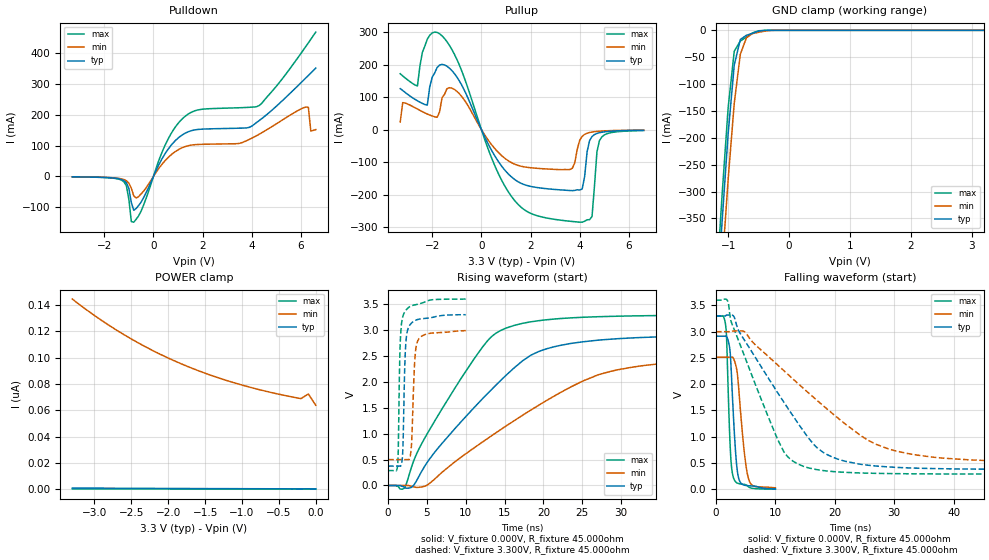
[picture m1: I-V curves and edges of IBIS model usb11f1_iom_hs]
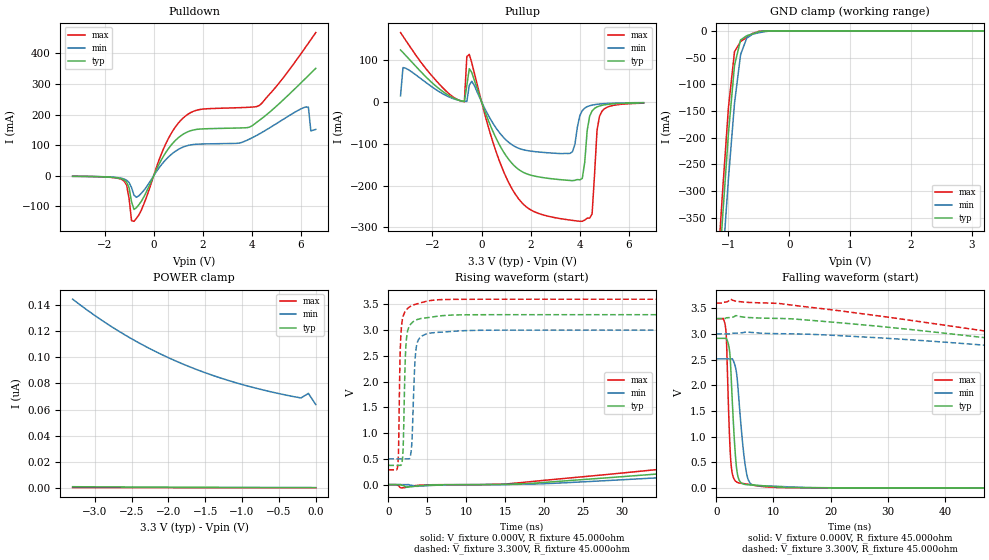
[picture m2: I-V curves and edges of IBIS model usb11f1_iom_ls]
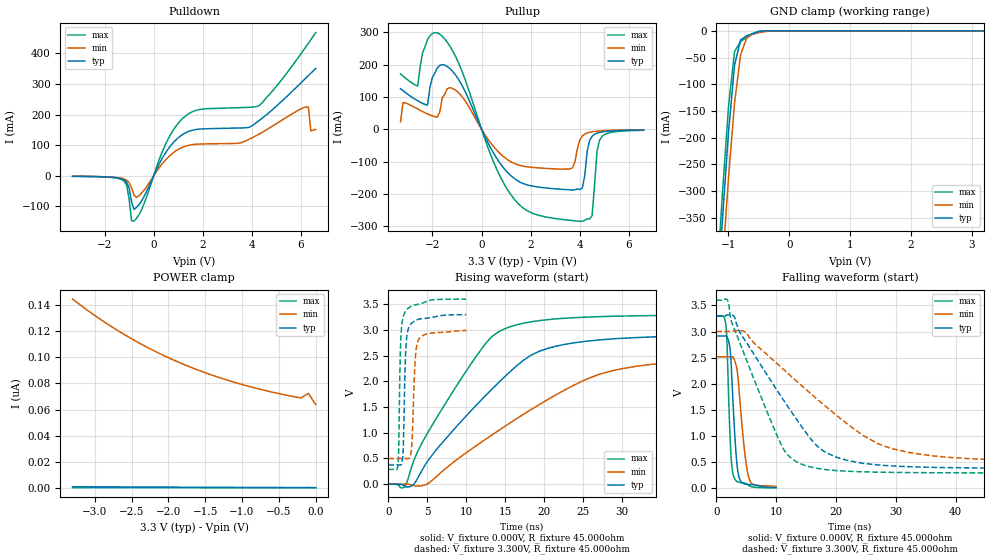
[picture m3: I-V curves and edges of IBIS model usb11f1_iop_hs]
[IBIS Ver]  4.0
[File Name]  lpc2929_lqfp144.ibs
[File Rev]  1.0
[Date]  Fri Oct 31 10:34:29 2008
[Source]  Package model is generic
[Notes]   IO models Rev 0.20 IBIS Model Design Automation Generation
[Copyright]  NXP Semiconductors 2008. All rights reserved.
[Disclaimer]
| NXP Semiconductors warrants and represents that the IBIS models
| identified herein are owned by NXP Semiconductors (NXP).  The
| models provided are not warranted as fully representing all of the
| operating characteristics and specifications of the semiconductor
| products to which the models relate.  Moreover, unless there is a
| signed, written agreement to the contrary, these models are furnished
| on an "as is" basis without support or warranty of any kind, either
| expressed or implied, regarding the use thereof, and NXP
| specifically disclaims all implied warranties of merchantability and
| fitness of the models for any purpose.
| NXP does not assume any liability arising out of the application
| or use of these IBIS models including infringement of patents and
| copyrights, nor does NXP convey any license under its patents and
| copyrights or the rights of others.
| NXP provides IBIS models as a service to our customers.  You and
| your company shall not distribute, convey, sell, or give these models
| to anyone else without receiving prior written permission from
| NXP.
[Component]   LPC29XX_LQFP144_01
[Manufacturer]  NXP
[Package]
|[Package Model]  LQFP144
|variable   typ   min   max
R_pkg   130.00m   123.00m   137.00m
L_pkg   8.30nH   7.50nH   9.20nH
C_pkg   1.00pF   0.80pF   1.30pF
| IMPORTANT NOTES:
| This model is valid for the following part types:
| LPC2929, LPC2927
| Signal names may be slightly different from the data
| sheet due to the 20 Char length limitation
[Pin]   signal_name   model_name   | comments
1 TDO bpats5thpept5v
2 P2.21 bpats5thpept5v
3 P0.24 bpats5thpept5v
4 P0.25 bpats5thpept5v
5 P0.26 bpats5thpept5v
6 P0.27 bpats5thpept5v
7 P0.28 bpats5thpept5v
8 P0.29 bpats5thpept5v
9 POWER_10 POWER
10 P2.22 bpats5thpept5v
11 P2.23 bpats5thpept5v
12 P3.6 bpats5thpept5v
13 P3.7 bpats5thpept5v
14 P0.30 bpats5thpept5v
15 P0.31 bpats5thpept5v
16 P2.24 bpats5thpept5v
17 P2.25 bpats5thpept5v
18 GND_21 POWER
19 USB1_IOP usb11f1_iop_ls
20 USB1_IOM usb11f1_iom_ls
21 POWER_26 POWER
22 POWER_27 POWER
23 GND_28 POWER
24 GND_30 POWER
25 P3_8 bpats5thpept5v
26 P3_9 bpats5thpept5v
27 P2_26 bpats5thpept5v
28 P2_27 bpats5thpept5v
29 P1.27 bpats5thpept5v
30 P1.26 bpats5thpept5v
31 POWER_48 POWER
32 P1.25 bpats5thpept5v
33 P1.24 bpats5thpept5v
34 P1.23 bpats5thpept5v
35 P1.22 bpats5thpept5v
36 TMS bpats5thpept5v
37 TCK bpats5thpept5v
38 P1.21 bpats5thpept5v
39 P1.20 bpats5thpept5v
40 P1.19 bpats5thpept5v
41 P1.18 bpats5thpept5v
42 P1.17 bpats5thpept5v
43 GNDE_62 POWER
44 P1.16 bpats5thpept5v
45 P2.0 bpats5thpept5v
46 P2.1 bpats5thpept5v
47 P3.10 bpats5thpept5v
48 P3.11 bpats5thpept5v
49 P1.15 bpats5thpept5v
50 P1.14 bpats5thpept5v
51 P1.13 bpats5thpept5v
52 P1.12 bpats5thpept5v
53 POWER_88 POWER
54 P2.2 bpats5thpept5v
55 P2.3 bpats5thpept5v
56 P1.11 bpats5thpept5v
57 P1.10 bpats5thpept5v
58 P3.12 bpats5thpept5v
59 GND_94 POWER
60 VDD_95 POWER
61 P3.13 bpats5thpept5v
62 P2.4 bpats5thpept5v
63 P2.5 bpats5thpept5v
64 P1.9 bpats5thpept5v
65 GNDE_100 POWER
66 P1.8 bpats5thpept5v
67 P1.7 bpats5thpept5v
68 P1.6 bpats5thpept5v
69 P2.6 bpats5thpept5v
70 P1.5 bpats5thpept5v
71 P1.4 bpats5thpept5v
72 TRSTN bpats5thpept5v
73 RSTN bpats5thpept5v
74 VSSA_OSC POWER
75 XOUT_OSC NC
76 XIN_OSC NC
77 VDDA_OSC POWER
78 VSSA_PLL POWER
79 P2.7 bpats5thpept5v
80 P3.14 bpats5thpept5v
81 P3.15 bpats5thpept5v
82 POWER_119 POWER
83 P2.8 bpats5thpept5v
84 P2.9 bpats5thpept5v
85 P1.3 bpats5thpept5v
86 P1.2 bpats5thpept5v
87 P1.1 bpats5thpept5v
88 GND_125 POWER
89 VDD_127 POWER
90 P1.0 bpats5thpept5v
91 P2.10 bpats5thpept5v
92 P2.11 bpats5thpept5v
93 P0.0 bpats5thpept5v
94 GNDE_134 POWER
95 P0.1 bpats5thpept5v
96 P0.2 bpats5thpept5v
97 P0.3 bpats5thpept5v
98 P3.0 bpats5thpept5v
99 P3.1 bpats5thpept5v
100 P2.12 bpats5thpept5v
101 P2.13 bpats5thpept5v
102 P0.4 bpats5thpept5v
103 P0.5 bpats5thpept5v
104 POWER_161 POWER
105 P0.6 bpats5thpept5v
106 P0.7 bpats5thpept5v
107 A3V3 POWER
108 JTAGSEL bpats5thpept5v
109 A5V POWER
110 VREFP NC
111 VREFN NC
112 P0.8 bpats5thpept5v
113 P0.9 bpats5thpept5v
114 P0.10 bpats5thpept5v
115 P0.11 bpats5thpept5v
116 P2.14 bpats5thpept5v
117 P2.15 bpats5thpept5v
118 P3.2 bpats5thpept5v
119 GNDE_178 POWER
120 P3.3 bpats5thpept5v
121 P0.12 bpats5thpept5v
122 P0.13 bpats5thpept5v
123 P0.14 bpats5thpept5v
124 P0.15 bpats5thpept5v
125 P0.16 bpats5thpept5v
126 P0.17 bpats5thpept5v
127 VDD_198 POWER
128 GND_199 POWER
129 P2.16 bpats5thpept5v
130 P2.17 bpats5thpept5v
131 POWER_202 POWER
132 P0.18 bpats5thpept5v
133 P0.19 bpats5thpept5v
134 P3.4 bpats5thpept5v
135 P3.5 bpats5thpept5v
136 P2.18 bpats5thpept5v
137 P2.19 bpats5thpept5v
138 P0.20 bpats5thpept5v
139 P0.21 bpats5thpept5v
140 P0.22 bpats5thpept5v
141 GNDE_212 POWER
142 P0.23 bpats5thpept5v
143 P2.20 bpats5thpept5v
144 TDI bpats5thpept5v
[Model Selector] bpats5thpept5v
bpats5thpept5v_p   Plain input Mode (p1=0, p2=1)
bpats5thpept5v_pd   Pull Down Mode   (p1=0, p2=0)
bpats5thpept5v_pu   Pull up   Mode   (p1=1, p2=1)
bpats5thpept5v_r   Repeater  Mode   (p1=1, p2=0)
[Model Selector] bpts5ptpht5v
bpts5ptpht5v_p_sh   Plain input Mode (p1=0, p2=1)
bpts5ptpht5v_p_sl   Plain input Mode (p1=0, p2=1)
bpts5ptpht5v_pd_sh   Pull Down Mode (p1=1, p2=1)
bpts5ptpht5v_pd_sl   Pull Down Mode (p1=1, p2=1)
bpts5ptpht5v_pu_sh   Pull Up Mode (p1=0, p2=0)
bpts5ptpht5v_pu_sl   Pull Up Mode (p1=0, p2=0)
bpts5ptpht5v_r_sh   Repeater Mode (p1=1, p2=0)
bpts5ptpht5v_r_sl   Repeater Mode (p1=1, p2=0)
| Models and submodels in the file (16): usb11f1_iom_hs (I/O), usb11f1_iom_ls (I/O), usb11f1_iop_hs (I/O), usb11f1_iop_ls (I/O), bpats5thpept5v_p (I/O), bpats5thpept5v_pd (I/O), bpats5thpept5v_pu (I/O), bpats5thpept5v_r (I/O), bpts5ptpht5v_p_sh (I/O), bpts5ptpht5v_p_sl (I/O), bpts5ptpht5v_pd_sh (I/O), bpts5ptpht5v_pd_sl (I/O), bpts5ptpht5v_pu_sh (I/O), bpts5ptpht5v_pu_sl (I/O), bpts5ptpht5v_r_sh (I/O), bpts5ptpht5v_r_sl (I/O)
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| usb11f1
|   Universal Serial Bus Pad
|   Revision 1.1 Specification
|   Programmable Single Ended Core Input
|   Forced Single Ended Low
|   Switchable between
|   - high speed output mode
|   - low speed output mode
|   - low/high speed input mode
| |   Rev 0.20 IBIS Model Design Automation Generation   |
| |   N O N - S I L I C O N   C O R R E L A T E D   |
| |   This IBIS [Model] is pre-Beta tactical support   |
| |  Note: this IBIS [Model] contains clamp curves generated   |
| |   through simulation which should not be relied upon   |
| Pccmos14 hliolib_nlm 4.0
|   0.18 um 3.3V pad library
|   six level metal
|   dual oxide
|   single threshold voltage
|   nominal line mixed supply
|   parasitic extracted netlists
| Process block c14
| High Speed Output Mode
[Model]   usb11f1_iom_hs | of usb11f1
Model_type   I/O
Polarity   Non-Inverting
Enable   Active-Low
|  Reciever Thresholds
Vinl   = 0.8V
Vinh   = 2.0V
| AC Test Load Conditions
Vref   = 0
Cref   = 0
Rref   = 1000000000
Vmeas   = 1.65
| [Process Range]   typical   min   max
| C_comp edge width   400.000ps   400.000ps   400.000ps
| C_comp Tstrobe   40.000fs   40.000fs   40.000fs
C_comp   3.752pF   3.496pF   4.045pF
[Temperature Range]   25   125   -40
[Voltage Range]   3.30V   3.00V   3.60V
[GND Clamp Reference]   0.00V   0.00V   0.00V
[Pulldown Reference]   0.00V   0.00V   0.00V
[POWER Clamp Reference]   3.30V   3.00V   3.60V
[Pullup Reference]   3.30V   3.00V   3.60V
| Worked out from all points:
|   slope of the pulldown table from 0 to 0.495 V, typ, clamps not added: 6.48 ohm
|   slope of the pullup table from 0 to 0.495 V, typ, clamps not added: 6.61 ohm
|   GND clamp passes 1 mA (typ) near -0.46 V on its own axis
|   rising waveform, V_fixture 0.000V, R_fixture 45.000ohm: 20-80 % time 11ns typ, 15.9ns min, 8.17ns max; typ from 0 V to 2.91 V
|   falling waveform, V_fixture 0.000V, R_fixture 45.000ohm: 20-80 % time 845ps typ, 1.21ns min, 607ps max; typ from 2.91 V to 0.006 V
|   rising waveform, V_fixture 3.300V, R_fixture 45.000ohm: 20-80 % time 320ps typ, 399ps min, 287ps max; typ from 0.374 V to 3.3 V
|   falling waveform, V_fixture 3.300V, R_fixture 45.000ohm: 20-80 % time 10.2ns typ, 15.5ns min, 6.95ns max; typ from 3.3 V to 0.374 V
[GND Clamp]
| ref voltage   0.00V   0.00V   0.00V
|   Voltage   I(typ)   I(min)   I(max)
-3.3V     -4.618A    -4.67A     -4.591A
-1.2V     -533.4mA   -616mA     -486.2mA
-1.1V     -356.1mA   -441.1mA   -306.9mA
-1V       -192.1mA   -277.1mA   -143.8mA
-900mV    -64.59mA   -135.6mA   -38.91mA
-800mV    -17.04mA   -44.51mA   -19.95mA
-700mV    -9.237mA   -13.86mA   -12.52mA
-600mV    -5.456mA   -6.064mA   -4.789mA
-500mV    -1.495mA   -3.666mA   -840.2uA
-300mV    -6.625uA   -179.7uA   -408.9nA
3.2V      293.2pA    68.89nA    105.6pA
[Power Clamp]   | Vtable = Vcc - Vpad
| ref voltage   3.30V   3.00V   3.60V
|   Voltage   I(typ)   I(min)   I(max)
-3.3V     1.005nA    144.5nA    354.7pA
-3V       911.2pA    132nA      335.1pA
-2.6V     800.8pA    117.4nA    309pA
-2.3V     727.5pA    108nA      289.6pA
-1.9V     640.7pA    97.15nA    263.8pA
-1.6V     582.9pA    90.25nA    244.5pA
-1.3V     530.6pA    84.3nA     225.3pA
-1V       483pA      79.18nA    206.1pA
-700mV    439.6pA    74.79nA    187pA
-200mV    377.6pA    68.89nA    155pA
-100mV    416.5pA    72.39nA    142.6pA
0V        319.1pA    63.83nA    125.6pA
[Pulldown]
| ref voltage   0.00V   0.00V   0.00V
|   Voltage   I(typ)   I(min)   I(max)
-3.3V     -1.652mA   -1.454mA   -1.796mA
-1.2V     -13.92mA   -10.45mA   -17.73mA
-1.1V     -21.12mA   -14.45mA   -30.61mA
-900mV    -85.23mA   -38.63mA   -146.6mA
-800mV    -110mA     -63.62mA   -148.7mA
500mV     77.03mA    53.28mA    105.7mA
1.1V      130.5mA    90.36mA    180.9mA
4.3V      181mA      136.8mA    229.8mA
6.2V      319.7mA    225.1mA    421.9mA
6.3V      327.6mA    224.1mA    433.3mA
6.4V      335.5mA    146.8mA    444.9mA
6.6V      351.2mA    151.8mA    468.2mA
[Pullup]   | Vtable = Vcc - Vpad
| ref voltage   3.30V   3.00V   3.60V
|   Voltage   I(typ)   I(min)   I(max)
-3.3V     125.8mA    23.2mA     171.5mA
-2.6V     88.3mA     62.98mA    134mA
-2.2V     74.98mA    47.7mA     277.9mA
-1.6V     200.3mA    97.67mA    288.3mA
-1V       161.8mA    117.7mA    216.4mA
900mV     -120mA     -85.3mA    -166.8mA
2.5V      -180.9mA   -120.7mA   -269.8mA
3.7V      -188.1mA   -119.1mA   -283mA
4.1V      -182.9mA   -20.96mA   -285.2mA
4.4V      -34.22mA   -9.287mA   -277.5mA
4.8V      -9.883mA   -5.195mA   -34.66mA
6.6V      -2.365mA   -1.804mA   -3.161mA
[Ramp]
R_load   = 60.000ohm
|   dV/dt(typ)   dV/dt(min)   dV/dt(max)
dV/dt_r   803.394mV/4.105ns   370.492mV/2.885ns   1.331V/4.905ns
dV/dt_f   843.371mV/4.620ns   360.067mV/3.240ns   1.540V/5.255ns
[Rising Waveform]  | cubic spline decimation from 16001 points
V_fixture   = 0.000V
R_fixture   = 45.000ohm
|   Time   V(typ)   V(min)   V(max)
0s        443.9pV    34.48nV    250.2pV
2.05ns    -28.68mV   9.864uV    -55.51mV
3.165ns   -16.71mV   -18.22mV   419.1mV
5.14ns    468.7mV    16.86mV    1.024V
12.03ns   1.653V     825.1mV    2.643V
16.32ns   2.281V     1.258V     3.093V
21.57ns   2.684V     1.741V     3.215V
26.99ns   2.804V     2.132V     3.257V
32.92ns   2.858V     2.315V     3.276V
80ns      2.912V     2.506V     3.295V
[Falling Waveform]  | cubic spline decimation from 2001 points
V_fixture   = 0.000V
R_fixture   = 45.000ohm
|   Time   V(typ)   V(min)   V(max)
0s        2.914V     2.514V     3.296V
1.65ns    2.919V     2.514V     3.102V
1.79ns    2.905V     2.514V     2.86V
2.415ns   2.567V     2.514V     760.7mV
2.935ns   1.397V     2.492V     222.4mV
3.365ns   607.8mV    2.348V     134.4mV
3.78ns    227.5mV    1.985V     109.9mV
4.655ns   81.21mV    824.9mV    94.37mV
5.45ns    66.93mV    210.5mV    47.53mV
10ns      6.197mV    27.24mV    1.84mV
[Rising Waveform]  | cubic spline decimation from 2001 points
V_fixture   = 3.300V
V_fixture_min = 3.000V
V_fixture_max = 3.600V
R_fixture   = 45.000ohm
|   Time   V(typ)   V(min)   V(max)
0s        373.7mV    499.4mV    287.7mV
1.215ns   373.7mV    499.4mV    375.2mV
1.575ns   374.2mV    499.5mV    2.78V
1.87ns    595mV      499.5mV    3.244V
2.065ns   1.779V     499.5mV    3.327V
2.355ns   2.862V     499.5mV    3.393V
2.96ns    3.126V     677.4mV    3.465V
3.43ns    3.18V      2.396V     3.486V
3.84ns    3.205V     2.798V     3.499V
10ns      3.296V     2.989V     3.598V
[Falling Waveform]  | cubic spline decimation from 16001 points
V_fixture   = 3.300V
V_fixture_min = 3.000V
V_fixture_max = 3.600V
R_fixture   = 45.000ohm
|   Time   V(typ)   V(min)   V(max)
0s        3.3V       3V         3.6V
1.96ns    3.316V     3V         3.585V
2.955ns   3.297V     3.013V     3.074V
4.81ns    2.836V     3V         2.532V
11.41ns   1.661V     2.26V      717.5mV
14.73ns   1.108V     1.92V      436.6mV
20.49ns   574.7mV    1.36V      330.4mV
25.63ns   457.1mV    931.8mV    306.2mV
31.99ns   408.5mV    686.3mV    295.4mV
80ns      374.5mV    503.6mV    287.9mV
| usb11f1
|   Universal Serial Bus Pad
|   Revision 1.1 Specification
|   Programmable Single Ended Core Input
|   Forced Single Ended Low
|   Switchable between
|   - high speed output mode
|   - low speed output mode
|   - low/high speed input mode
| |   Rev 0.20 IBIS Model Design Automation Generation   |
| |   N O N - S I L I C O N   C O R R E L A T E D   |
| |   This IBIS [Model] is pre-Beta tactical support   |
| |  Note: this IBIS [Model] contains clamp curves generated   |
| |   through simulation which should not be relied upon   |
| Pccmos14 hliolib_nlm 4.0
|   0.18 um 3.3V pad library
|   six level metal
|   dual oxide
|   single threshold voltage
|   nominal line mixed supply
|   parasitic extracted netlists
| Process block c14
| Low Speed Output Mode
[Model]   usb11f1_iom_ls | of usb11f1
Model_type   I/O
Polarity   Non-Inverting
Enable   Active-Low
|  Reciever Thresholds
Vinl   = 0.8V
Vinh   = 2.0V
| AC Test Load Conditions
Vref   = 0
Cref   = 0
Rref   = 1000000000
Vmeas   = 1.65
| [Process Range]   typical   min   max
| C_comp edge width   400.000ps   400.000ps   400.000ps
| C_comp Tstrobe   40.000fs   40.000fs   40.000fs
C_comp   3.752pF   3.496pF   4.045pF
[Temperature Range]   25   125   -40
[Voltage Range]   3.30V   3.00V   3.60V
[GND Clamp Reference]   0.00V   0.00V   0.00V
[Pulldown Reference]   0.00V   0.00V   0.00V
[POWER Clamp Reference]   3.30V   3.00V   3.60V
[Pullup Reference]   3.30V   3.00V   3.60V
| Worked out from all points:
|   slope of the pulldown table from 0 to 0.495 V, typ, clamps not added: 6.48 ohm
|   slope of the pullup table from 0 to 0.495 V, typ, clamps not added: 6.61 ohm
|   GND clamp passes 1 mA (typ) near -0.46 V on its own axis
|   rising waveform, V_fixture 0.000V, R_fixture 45.000ohm: 20-80 % time 151ns typ, 180ns min, 132ns max; typ from 0 V to 2.91 V
|   falling waveform, V_fixture 0.000V, R_fixture 45.000ohm: 20-80 % time 850ps typ, 1.23ns min, 609ps max; typ from 2.91 V to 0 V
|   rising waveform, V_fixture 3.300V, R_fixture 45.000ohm: 20-80 % time 318ps typ, 398ps min, 284ps max; typ from 0.374 V to 3.3 V
|   falling waveform, V_fixture 3.300V, R_fixture 45.000ohm: 20-80 % time 156ns typ, 194ns min, 133ns max; typ from 3.3 V to 0.38 V
[GND Clamp]
| ref voltage   0.00V   0.00V   0.00V
|   Voltage   I(typ)   I(min)   I(max)
-3.3V     -4.618A    -4.67A     -4.591A
-1.2V     -533.4mA   -616mA     -486.2mA
-1.1V     -356.1mA   -441.1mA   -306.9mA
-1V       -192.1mA   -277.1mA   -143.8mA
-900mV    -64.59mA   -135.6mA   -38.91mA
-800mV    -17.04mA   -44.51mA   -19.95mA
-700mV    -9.237mA   -13.86mA   -12.52mA
-600mV    -5.456mA   -6.064mA   -4.789mA
-500mV    -1.495mA   -3.666mA   -840.2uA
-300mV    -6.625uA   -179.7uA   -408.9nA
3.2V      293.2pA    68.89nA    105.6pA
[Power Clamp]   | Vtable = Vcc - Vpad
| ref voltage   3.30V   3.00V   3.60V
|   Voltage   I(typ)   I(min)   I(max)
-3.3V     1.005nA    144.5nA    354.7pA
-3V       911.2pA    132nA      335.1pA
-2.6V     800.8pA    117.4nA    309pA
-2.3V     727.5pA    108nA      289.6pA
-1.9V     640.7pA    97.15nA    263.8pA
-1.6V     582.9pA    90.25nA    244.5pA
-1.3V     530.6pA    84.3nA     225.3pA
-1V       483pA      79.18nA    206.1pA
-700mV    439.6pA    74.79nA    187pA
-200mV    377.6pA    68.89nA    155pA
-100mV    416.5pA    72.39nA    142.6pA
0V        319.1pA    63.83nA    125.6pA
[Pulldown]
| ref voltage   0.00V   0.00V   0.00V
|   Voltage   I(typ)   I(min)   I(max)
-3.3V     -1.652mA   -1.454mA   -1.796mA
-1.2V     -13.92mA   -10.45mA   -17.73mA
-1.1V     -21.12mA   -14.45mA   -30.61mA
-900mV    -85.23mA   -38.63mA   -146.6mA
-800mV    -110mA     -63.62mA   -148.7mA
500mV     77.03mA    53.28mA    105.7mA
1.1V      130.5mA    90.36mA    180.9mA
4.3V      181mA      136.8mA    229.8mA
6.2V      319.7mA    225.1mA    421.9mA
6.3V      327.6mA    224.1mA    433.3mA
6.4V      335.5mA    146.8mA    444.9mA
6.6V      351.2mA    151.8mA    468.2mA
[Pullup]   | Vtable = Vcc - Vpad
| ref voltage   3.30V   3.00V   3.60V
|   Voltage   I(typ)   I(min)   I(max)
-3.3V     123.9mA    14.28mA    165.4mA
-3.2V     117.8mA    81.84mA    156.7mA
-800mV    1.807mA    2.206mA    1.368mA
-500mV    79.1mA     39.57mA    113.5mA
1V        -129mA     -91.21mA   -180.1mA
2.5V      -180.9mA   -120.7mA   -269.8mA
3.7V      -188.1mA   -119.1mA   -283mA
4.1V      -182.9mA   -20.96mA   -285.2mA
4.4V      -34.22mA   -9.287mA   -277.5mA
4.5V      -21.68mA   -7.778mA   -267.6mA
4.8V      -9.883mA   -5.195mA   -34.66mA
6.6V      -2.365mA   -1.804mA   -3.161mA
[Ramp]
R_load   = 60.000ohm
|   dV/dt(typ)   dV/dt(min)   dV/dt(max)
dV/dt_r   621.133mV/49.000ns   449.857mV/47.650ns   797.798mV/50.350ns
dV/dt_f   625.100mV/49.850ns   419.096mV/47.300ns   836.278mV/52.000ns
[Rising Waveform]  | cubic spline decimation from 16001 points
V_fixture   = 0.000V
R_fixture   = 45.000ohm
|   Time   V(typ)   V(min)   V(max)
0s        443.9pV    34.49nV    250.2pV
1.75ns    -12.65mV   2.275uV    -62.94mV
15.6ns    5.793mV    2.484mV    18.34mV
130.2ns   1.408V     1.033V     1.795V
182.8ns   2.006V     1.49V      2.541V
215.3ns   2.324V     1.742V     2.891V
240.8ns   2.515V     1.918V     3.033V
308.5ns   2.738V     2.227V     3.184V
402.4ns   2.838V     2.384V     3.248V
800ns     2.907V     2.501V     3.292V
[Falling Waveform]  | cubic spline decimation from 2001 points
V_fixture   = 0.000V
R_fixture   = 45.000ohm
|   Time   V(typ)   V(min)   V(max)
0s        2.914V     2.514V     3.296V
1.65ns    2.918V     2.514V     3.099V
1.8ns     2.902V     2.514V     2.824V
2.25ns    2.726V     2.514V     1.203V
2.75ns    1.81V      2.518V     313.5mV
3.35ns    628.5mV    2.352V     134.1mV
3.85ns    197.5mV    1.878V     99.95mV
5.3ns     62.15mV    280.7mV    75.31mV
6.75ns    52.95mV    48.63mV    46.78mV
100ns     89.79uV    122.2uV    67.53uV
[Rising Waveform]  | cubic spline decimation from 2001 points
V_fixture   = 3.300V
V_fixture_min = 3.000V
V_fixture_max = 3.600V
R_fixture   = 45.000ohm
|   Time   V(typ)   V(min)   V(max)
0s        373.7mV    499.4mV    287.7mV
1.25ns    373.7mV    499.5mV    440.2mV
1.55ns    374.8mV    499.5mV    2.698V
1.85ns    558.6mV    499.5mV    3.237V
2.15ns    2.321V     499.5mV    3.356V
2.4ns     2.919V     499.6mV    3.406V
3ns       3.136V     762.4mV    3.473V
3.6ns     3.197V     2.674V     3.505V
4.85ns    3.237V     2.922V     3.556V
100ns     3.3V       3V         3.6V
[Falling Waveform]  | cubic spline decimation from 16001 points
V_fixture   = 3.300V
V_fixture_min = 3.000V
V_fixture_max = 3.600V
R_fixture   = 45.000ohm
|   Time   V(typ)   V(min)   V(max)
0s        3.3V       3V         3.6V
2.45ns    3.319V     3V         3.678V
28.5ns    3.148V     2.924V     3.35V
114.5ns   2.081V     2.172V     1.981V
188.3ns   1.259V     1.566V     937.8mV
232.7ns   858.8mV    1.248V     557.2mV
289.8ns   591.2mV    921.5mV    405.8mV
389.9ns   453.5mV    659.5mV    332.3mV
557.6ns   398mV      548.8mV    301.5mV
800ns     380mV      513mV      291.2mV
| usb11f1
|   Universal Serial Bus Pad
|   Revision 1.1 Specification
|   Programmable Single Ended Core Input
|   Forced Single Ended Low
|   Switchable between
|   - high speed output mode
|   - low speed output mode
|   - low/high speed input mode
| |   Rev 0.20 IBIS Model Design Automation Generation   |
| |   N O N - S I L I C O N   C O R R E L A T E D   |
| |   This IBIS [Model] is pre-Beta tactical support   |
| |  Note: this IBIS [Model] contains clamp curves generated   |
| |   through simulation which should not be relied upon   |
| Pccmos14 hliolib_nlm 4.0
|   0.18 um 3.3V pad library
|   six level metal
|   dual oxide
|   single threshold voltage
|   nominal line mixed supply
|   parasitic extracted netlists
| Process block c14
| High Speed Output Mode
[Model]   usb11f1_iop_hs | of usb11f1
Model_type   I/O
Polarity   Non-Inverting
Enable   Active-Low
|  Reciever Thresholds
Vinl   = 0.8V
Vinh   = 2.0V
| AC Test Load Conditions
Vref   = 0
Cref   = 0
Rref   = 1000000000
Vmeas   = 1.65
| [Process Range]   typical   min   max
| C_comp edge width   400.000ps   400.000ps   400.000ps
| C_comp Tstrobe   40.000fs   40.000fs   40.000fs
C_comp   3.752pF   3.496pF   4.045pF
[Temperature Range]   25   125   -40
[Voltage Range]   3.30V   3.00V   3.60V
[GND Clamp Reference]   0.00V   0.00V   0.00V
[Pulldown Reference]   0.00V   0.00V   0.00V
[POWER Clamp Reference]   3.30V   3.00V   3.60V
[Pullup Reference]   3.30V   3.00V   3.60V
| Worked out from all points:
|   slope of the pulldown table from 0 to 0.495 V, typ, clamps not added: 6.48 ohm
|   slope of the pullup table from 0 to 0.495 V, typ, clamps not added: 6.61 ohm
|   GND clamp passes 1 mA (typ) near -0.46 V on its own axis
|   rising waveform, V_fixture 0.000V, R_fixture 45.000ohm: 20-80 % time 11ns typ, 15.9ns min, 8.17ns max; typ from 0 V to 2.91 V
|   falling waveform, V_fixture 0.000V, R_fixture 45.000ohm: 20-80 % time 847ps typ, 1.21ns min, 606ps max; typ from 2.91 V to 0.006 V
|   rising waveform, V_fixture 3.300V, R_fixture 45.000ohm: 20-80 % time 321ps typ, 402ps min, 285ps max; typ from 0.374 V to 3.3 V
|   falling waveform, V_fixture 3.300V, R_fixture 45.000ohm: 20-80 % time 10.2ns typ, 15.5ns min, 6.95ns max; typ from 3.3 V to 0.374 V
[GND Clamp]
| ref voltage   0.00V   0.00V   0.00V
|   Voltage   I(typ)   I(min)   I(max)
-3.3V     -4.618A    -4.67A     -4.591A
-1.2V     -533.4mA   -616mA     -486.2mA
-1.1V     -356.1mA   -441.1mA   -306.9mA
-1V       -192.1mA   -277.1mA   -143.8mA
-900mV    -64.59mA   -135.6mA   -38.91mA
-800mV    -17.04mA   -44.51mA   -19.95mA
-700mV    -9.237mA   -13.86mA   -12.52mA
-600mV    -5.456mA   -6.064mA   -4.789mA
-500mV    -1.495mA   -3.666mA   -840.2uA
-300mV    -6.625uA   -179.7uA   -408.9nA
3.2V      293.2pA    68.89nA    105.6pA
[Power Clamp]   | Vtable = Vcc - Vpad
| ref voltage   3.30V   3.00V   3.60V
|   Voltage   I(typ)   I(min)   I(max)
-3.3V     1.005nA    144.5nA    354.7pA
-3V       911.2pA    132nA      335.1pA
-2.6V     800.8pA    117.4nA    309pA
-2.3V     727.5pA    108nA      289.6pA
-1.9V     640.7pA    97.15nA    263.8pA
-1.6V     582.9pA    90.25nA    244.5pA
-1.3V     530.6pA    84.3nA     225.3pA
-1V       483pA      79.18nA    206.1pA
-700mV    439.6pA    74.79nA    187pA
-200mV    377.6pA    68.89nA    155pA
-100mV    416.5pA    72.39nA    142.6pA
0V        319.1pA    63.83nA    125.6pA
[Pulldown]
| ref voltage   0.00V   0.00V   0.00V
|   Voltage   I(typ)   I(min)   I(max)
-3.3V     -1.652mA   -1.454mA   -1.796mA
-1.2V     -13.92mA   -10.45mA   -17.73mA
-1.1V     -21.12mA   -14.45mA   -30.61mA
-900mV    -85.23mA   -38.63mA   -146.6mA
-800mV    -110mA     -63.62mA   -148.7mA
500mV     77.03mA    53.28mA    105.7mA
1.1V      130.5mA    90.36mA    180.9mA
4.3V      181mA      136.8mA    229.8mA
6.2V      319.7mA    225.1mA    421.9mA
6.3V      327.6mA    224.1mA    433.3mA
6.4V      335.5mA    146.8mA    444.9mA
6.6V      351.2mA    151.8mA    468.2mA
[Pullup]   | Vtable = Vcc - Vpad
| ref voltage   3.30V   3.00V   3.60V
|   Voltage   I(typ)   I(min)   I(max)
-3.3V     125.8mA    23.2mA     171.5mA
-2.6V     88.3mA     62.98mA    134mA
-2.2V     74.98mA    47.7mA     277.9mA
-1.6V     200.3mA    97.67mA    288.3mA
-1V       161.8mA    117.7mA    216.4mA
900mV     -120mA     -85.3mA    -166.8mA
2.5V      -180.9mA   -120.7mA   -269.8mA
3.7V      -188.1mA   -119.1mA   -283mA
4.1V      -182.9mA   -20.96mA   -285.2mA
4.4V      -34.22mA   -9.287mA   -277.5mA
4.8V      -9.883mA   -5.195mA   -34.66mA
6.6V      -2.365mA   -1.804mA   -3.161mA
[Ramp]
R_load   = 60.000ohm
|   dV/dt(typ)   dV/dt(min)   dV/dt(max)
dV/dt_r   802.872mV/4.105ns   370.430mV/2.890ns   1.330V/4.895ns
dV/dt_f   847.049mV/4.645ns   363.155mV/3.270ns   1.544V/5.270ns
[Rising Waveform]  | cubic spline decimation from 16001 points
V_fixture   = 0.000V
R_fixture   = 45.000ohm
|   Time   V(typ)   V(min)   V(max)
0s        443.9pV    34.48nV    250.2pV
2.065ns   -29.58mV   -1.03uV    -55.15mV
3.17ns    -16.87mV   -18.22mV   416.1mV
5.21ns    482.5mV    23.6mV     1.039V
12.08ns   1.661V     830.7mV    2.652V
16.39ns   2.289V     1.265V     3.095V
21.33ns   2.675V     1.719V     3.211V
26.95ns   2.803V     2.13V      3.257V
32.18ns   2.853V     2.3V       3.275V
80ns      2.912V     2.506V     3.295V
[Falling Waveform]  | cubic spline decimation from 2001 points
V_fixture   = 0.000V
R_fixture   = 45.000ohm
|   Time   V(typ)   V(min)   V(max)
0s        2.914V     2.514V     3.296V
1.64ns    2.92V      2.514V     3.086V
1.765ns   2.904V     2.514V     2.86V
2.38ns    2.57V      2.514V     783.4mV
2.935ns   1.326V     2.481V     213.7mV
3.41ns    505.1mV    2.301V     127.8mV
3.77ns    217.1mV    1.933V     109.5mV
4.66ns    79.74mV    768.8mV    93.98mV
5.445ns   66.7mV     193.7mV    45.74mV
10ns      6.095mV    26.73mV    1.823mV
[Rising Waveform]  | cubic spline decimation from 2001 points
V_fixture   = 3.300V
V_fixture_min = 3.000V
V_fixture_max = 3.600V
R_fixture   = 45.000ohm
|   Time   V(typ)   V(min)   V(max)
0s        373.7mV    499.4mV    287.7mV
1.245ns   373.7mV    499.4mV    398.8mV
1.58ns    374.4mV    499.5mV    2.748V
1.88ns    599.6mV    499.5mV    3.241V
2.075ns   1.793V     499.5mV    3.326V
2.365ns   2.864V     499.5mV    3.393V
2.965ns   3.125V     677.1mV    3.464V
3.435ns   3.18V      2.395V     3.485V
3.815ns   3.203V     2.788V     3.498V
10ns      3.296V     2.989V     3.598V
[Falling Waveform]  | cubic spline decimation from 16001 points
V_fixture   = 3.300V
V_fixture_min = 3.000V
V_fixture_max = 3.600V
R_fixture   = 45.000ohm
|   Time   V(typ)   V(min)   V(max)
0s        3.3V       3V         3.6V
1.905ns   3.316V     3V         3.592V
2.51ns    3.319V     3V         3.198V
5.015ns   2.793V     2.974V     2.463V
11.14ns   1.702V     2.283V     764.9mV
14.69ns   1.108V     1.918V     436.9mV
20.36ns   578.2mV    1.367V     331.2mV
27ns      441.4mV    850.1mV    302.8mV
32.03ns   408.2mV    684.4mV    295.3mV
80ns      374.5mV    503.6mV    287.9mV
